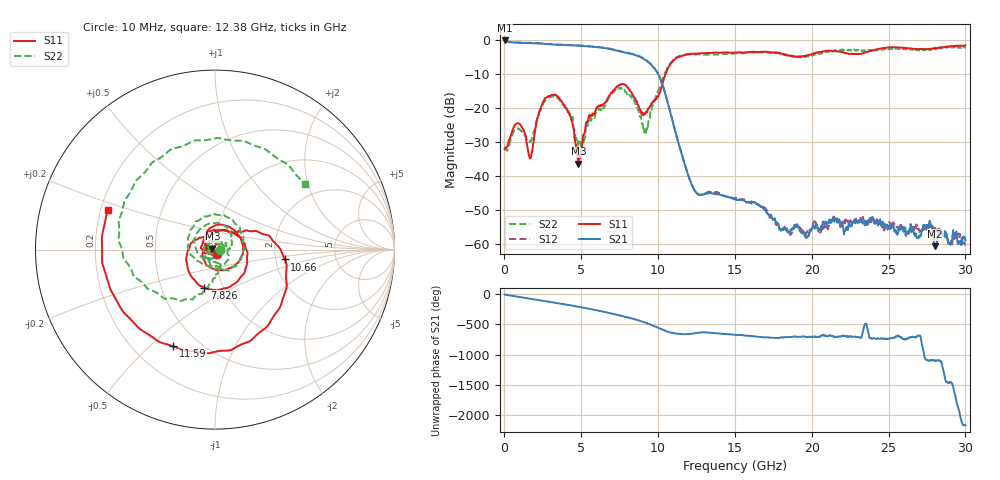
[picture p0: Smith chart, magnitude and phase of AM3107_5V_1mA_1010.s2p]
# Hz S DB R 50.0
!freq dBS11 angS11 dBS21 angS21 dBS12 angS12 dBS22 angS22
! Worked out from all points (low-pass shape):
!   1601 points, 10 MHz to 30 GHz, reference 50 ohm
!   highest |S21| = -0.09 dB at 10 MHz (marker M1); lowest = -60.7 dB at 28.03 GHz (marker M2)
!   |S21| within 3 dB of the highest: start of sweep to 7.323 GHz
!   lowest |S11| = -36.4 dB at 4.808 GHz (marker M3), VSWR 1.03, Z = 48.6 + j0.433 ohm
!   |S11| at or under -10 dB: start of sweep to 10.48 GHz
!   |S22| runs from -32.6 to -1.8 dB; largest |S21 - S12| = 0.011
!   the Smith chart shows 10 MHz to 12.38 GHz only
!   S11 on the Smith chart (normalised r, x): 10 MHz: 1.02, -0.05; 7.826 GHz: 0.81, -0.36; 10.66 GHz: 2.25, -0.29; 11.59 GHz: 0.36, -0.59; 12.38 GHz: 0.23, +0.17
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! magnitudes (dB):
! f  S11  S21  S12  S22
! 10 MHz  -32.1  -0.1  -0.1  -31.3
! 891 MHz  -24.5  -0.8  -0.7  -26.0
! 1.697 GHz  -34.7  -0.9  -0.8  -29.9
! 2.39 GHz  -19.5  -1.0  -1.0  -20.0
! 3.215 GHz  -16.1  -1.3  -1.2  -16.4
! 4.265 GHz  -22.2  -1.5  -1.4  -21.8
! 4.808 GHz  -36.4  -1.6  -1.5  -29.5
! 5.015 GHz  -31.9  -1.7  -1.6  -31.5
! 5.464 GHz  -23.1  -1.9  -1.7  -23.9
! 7.826 GHz  -13.1  -3.6  -3.5  -14.9
! 9.176 GHz  -21.6  -5.8  -5.7  -27.9
! 10.02 GHz  -16.5  -10.2  -10.1  -14.8
! 10.66 GHz  -8.1  -18.9  -18.8  -8.0
! 11.59 GHz  -4.6  -34.5  -34.4  -4.5
! 12.38 GHz  -3.9  -44.3  -44.4  -4.1
! 15.01 GHz  -3.7  -46.9  -46.6  -3.8
! 18.55 GHz  -4.6  -56.5  -57.7  -4.4
! 20.01 GHz  -4.1  -55.7  -55.4  -4.6
! 25.01 GHz  -2.1  -55.4  -54.9  -2.6
! 27.66 GHz  -2.6  -53.6  -55.6  -2.9
! 28.03 GHz  -2.4  -60.7  -55.3  -2.6
! 30 GHz  -1.5  -59.0  -60.4  -1.9
